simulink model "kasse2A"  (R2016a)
settings: Solver=FixedStepDiscrete  StartTime=0.0  StopTime=100  FixedStep=0.001  RelTol=1e-3
undefined symbols (not defined in the file or in its folder): tAb, z0
libraries: simulink x2

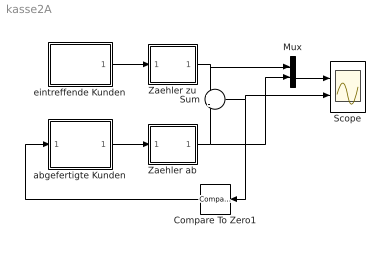
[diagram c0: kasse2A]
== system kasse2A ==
  Compare To Zero1 : simulink/Logic and Bit Operations/Compare To Zero  relop=<=  OutDataTypeStr=uint8
  Mux : Mux  Inputs=2
  Scope : Scope  NumInputPorts=2
  Sum : Sum  Inputs=+|-
  Zaehler ab : Subsystem
  Zaehler zu : Subsystem
  abgefertigte Kunden : Subsystem
  eintreffende Kunden : Subsystem
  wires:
  Zaehler zu/1(Out) -> Sum/1, Mux/1
  eintreffende Kunden/1(Out1) -> Zaehler zu/1(In)
  abgefertigte Kunden/1(Out) -> Zaehler ab/1(In)
  Zaehler ab/1(Out) -> Sum/2, Mux/2
  Sum/1 -> Compare To Zero1/1, Scope/2
  Compare To Zero1/1 -> abgefertigte Kunden/1(In1)
  Mux/1 -> Scope/1

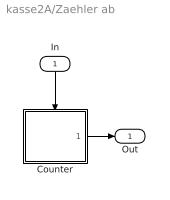
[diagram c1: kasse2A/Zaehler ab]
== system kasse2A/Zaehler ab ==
  In : Inport
  Counter : Subsystem
  Out : Outport
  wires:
  Counter/1(Out) -> Out/1
  In/1 -> Counter/Trigger

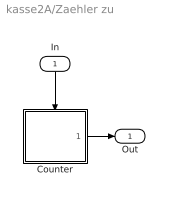
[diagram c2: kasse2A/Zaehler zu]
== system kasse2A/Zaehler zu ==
  In : Inport
  Counter : Subsystem
  Out : Outport
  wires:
  Counter/1(Out) -> Out/1
  In/1 -> Counter/Trigger

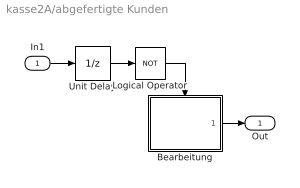
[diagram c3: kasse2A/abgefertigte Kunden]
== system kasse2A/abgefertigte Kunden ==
  In1 : Inport
  Bearbeitung : Subsystem
  Logical Operator : Logic  Operator=NOT  AllPortsSameDT=off  OutDataTypeStr=boolean
  Unit Delay : UnitDelay  SampleTime=-1
  Out : Outport
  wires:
  Logical Operator/1 -> Bearbeitung/Enable
  Unit Delay/1 -> Logical Operator/1
  In1/1 -> Unit Delay/1
  Bearbeitung/1(Out) -> Out/1

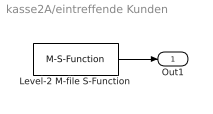
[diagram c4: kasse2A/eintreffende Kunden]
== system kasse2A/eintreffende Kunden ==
  Level-2 M-file S-Function : M-S-Function  FunctionName=sfun_poisson  Parameters=lambda
  Out1 : Outport
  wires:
  Level-2 M-file S-Function/1 -> Out1/1

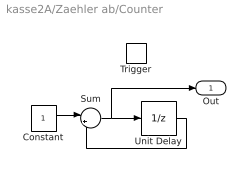
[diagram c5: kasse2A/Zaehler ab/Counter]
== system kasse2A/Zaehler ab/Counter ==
  Trigger : TriggerPort  TriggerType=falling  VariantControl=Variant
  Constant : Constant
  Sum : Sum  Inputs=|++
  Unit Delay : UnitDelay  InitialCondition=z0  SampleTime=-1
  Out : Outport  InitialOutput=z0
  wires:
  Constant/1 -> Sum/1
  Sum/1 -> Unit Delay/1, Out/1
  Unit Delay/1 -> Sum/2

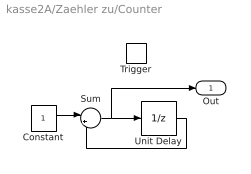
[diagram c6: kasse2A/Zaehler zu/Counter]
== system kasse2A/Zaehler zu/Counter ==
  Trigger : TriggerPort  TriggerType=falling  VariantControl=Variant
  Constant : Constant
  Sum : Sum  Inputs=|++
  Unit Delay : UnitDelay  InitialCondition=z0  SampleTime=-1
  Out : Outport  InitialOutput=z0
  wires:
  Constant/1 -> Sum/1
  Sum/1 -> Unit Delay/1, Out/1
  Unit Delay/1 -> Sum/2

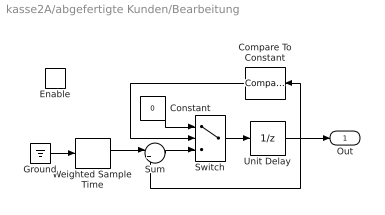
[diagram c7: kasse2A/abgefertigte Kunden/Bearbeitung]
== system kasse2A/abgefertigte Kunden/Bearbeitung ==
  Enable : EnablePort  StatesWhenEnabling=reset
  Compare To Constant : simulink/Logic and Bit Operations/Compare To Constant  SystemSampleTime=-1  relop=>=  const=tAb  LogicOutDataTypeMode=uint8
  Constant : Constant  Value=0
  Ground : Ground
  Sum : Sum  Inputs=|++
  Switch : Switch  Threshold=1
  Unit Delay : UnitDelay  SampleTime=-1
  Weighted Sample Time : SampleTimeMath  TsampMathOp=Ts Only  weightValue=1
  Out : Outport  OutputWhenDisabled=reset  InitialOutput=0
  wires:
  Unit Delay/1 -> Out/1, Sum/2, Compare To Constant/1
  Ground/1 -> Weighted Sample Time/1
  Weighted Sample Time/1 -> Sum/1
  Sum/1 -> Switch/3
  Switch/1 -> Unit Delay/1
  Constant/1 -> Switch/1
  Compare To Constant/1 -> Switch/2
